(* Logix 5000 AddOnInstructionDefinition export Banner_LTF_Param_v4; software revision 33.00; part 3 of 3 *)
(* tags used below, declared in another part *)
   LTF : Banner_LTF_v4;
   Port_Data : Banner_IOL_Port_v4;
   Port : DINT;
   Local_Control : DINT;
   Command_Being_Processed : BOOL;
   Update_Archive : BOOL;
   Index_Write_Inprocess : INT;
   Inprocess_Index : DINT;
(* Banner_LTF_Param_v4, continued *)

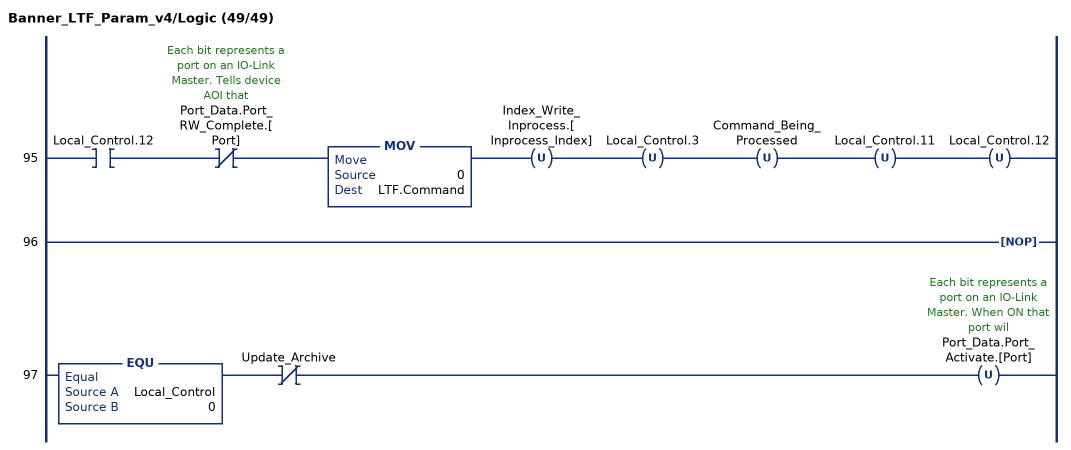
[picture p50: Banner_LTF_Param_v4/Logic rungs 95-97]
   95: XIC(Local_Control.12)XIO(Port_Data.Port_RW_Complete.[Port])MOV(0,LTF.Command)OTU(Index_Write_Inprocess.[Inprocess_Index])OTU(Local_Control.3)OTU(Command_Being_Processed)OTU(Local_Control.11)OTU(Local_Control.12);
   96: NOP();
   97: EQU(Local_Control,0)XIO(Update_Archive)OTU(Port_Data.Port_Activate.[Port]);
END_ROUTINE
END_ADD_ON_INSTRUCTION
